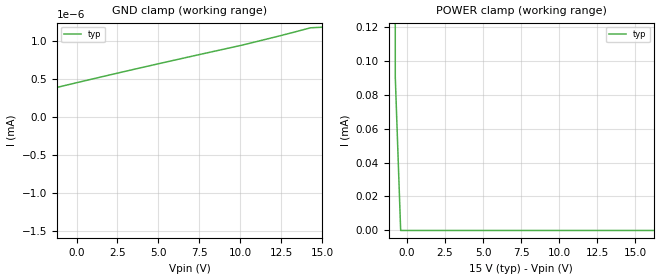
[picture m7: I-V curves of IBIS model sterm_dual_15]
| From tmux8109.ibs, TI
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| sterm_dual_15
[Model]   sterm_dual_15
Model_type   Terminator
|   typ   min   max
C_comp   4.014581e-12   NA   NA
[Voltage Range]   15   NA   NA
[Temperature Range]   27   NA   NA
[Power Clamp Reference]   15   NA   NA
[GND Clamp Reference]   0   NA   NA
[GND Clamp]
|   Voltage   I(typ)   I(min)   I(max)
-20V      -1.133A    NA         NA
-15.4V    -38.2nA    NA         NA
-15.05V   -269.4pA   NA         NA
-11.87V   -146pA     NA         NA
-9.394V   -33.74pA   NA         NA
1.919V    550.4pA    NA         NA
10.05V    946.3pA    NA         NA
14.29V    1.178nA    NA         NA
15V       1.185nA    NA         NA
[POWER Clamp]
|   Voltage   I(typ)   I(min)   I(max)
-5V       744mA      NA         NA
-1.111V   26.13mA    NA         NA
-757.6mV  90.5uA     NA         NA
-404mV    1.549nA    NA         NA
30V       -267.4pA   NA         NA
